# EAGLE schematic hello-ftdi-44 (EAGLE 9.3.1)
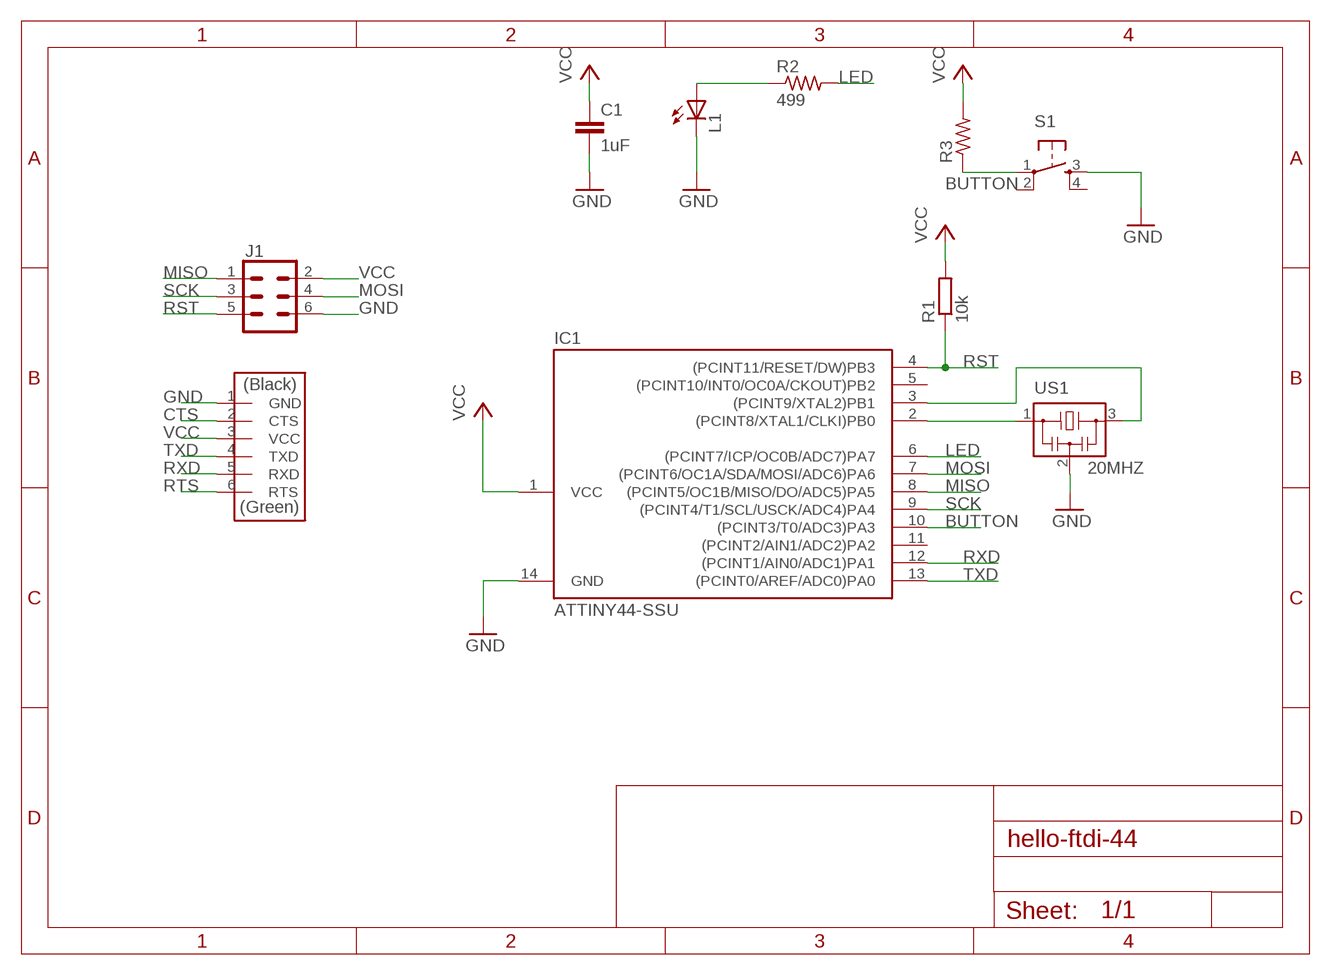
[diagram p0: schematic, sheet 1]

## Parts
C1  1uF  C-EUC1206  [C1206]
IC1  ATTINY44-SSU  [SOIC14]
J1  CONN_03X2SMT  [2X3_SMT_POSTS]
J2  FTDI-SMD-HEADER  [1X06SMD]
L1  LEDFAB1206  [LED1206FAB]
R1  10k  R-EU_M1206  [M1206]
R2  499  RES-US1206  [R1206]
R3  RES-US1206  [R1206]
S1  6MM_SWITCH6MM_SWITCH  [6MM_SWITCH]
US1  20MHZ  RESONATOR  [EFOBM]

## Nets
BUTTON: IC1.10((PCINT3/T0/ADC3)PA3) R3.1 S1.1(P)
CTS: J2.2(CTS)
GND: C1.2 IC1.14(GND) J1.6 J2.1(GND) L1.2(C) S1.3(S) US1.2
LED: IC1.6((PCINT7/ICP/OC0B/ADC7)PA7) R2.2
MISO: IC1.8((PCINT5/OC1B/MISO/DO/ADC5)PA5) J1.1
MOSI: IC1.7((PCINT6/OC1A/SDA/MOSI/ADC6)PA6) J1.4
N$1: L1.1(A) R2.1
N$7: IC1.2((PCINT8/XTAL1/CLKI)PB0) US1.1
N$8: IC1.3((PCINT9/XTAL2)PB1) US1.3
RST: IC1.4((PCINT11/RESET/DW)PB3) J1.5 R1.1
RTS: J2.6(RTS)
RXD: IC1.12((PCINT1/AIN0/ADC1)PA1) J2.5(RXD)
SCK: IC1.9((PCINT4/T1/SCL/USCK/ADC4)PA4) J1.3
TXD: IC1.13((PCINT0/AREF/ADC0)PA0) J2.4(TXD)
VCC: C1.1 IC1.1(VCC) J1.2 J2.3(VCC) R1.2 R3.2
Unconnected: IC1.5((PCINT10/INT0/OC0A/CKOUT)PB2) IC1.11((PCINT2/AIN1/ADC2)PA2) S1.2(P1) S1.4(S1)

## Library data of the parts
C1 = rcl:C-EU: CAPACITOR, European symbol
IC1 = fab:ATTINY44
J1 = SparkFun-Connectors:CONN_03X2: Multi connection point. Often used as Generic Header-pin footprint for 0.1 inch spaced/style header connections You can populate with any combo of single row headers, but if you'd like an exact match, check these: Header - 2x3 (Male, 0.1") (PRT-12807) Header - 2x3 (Female, 0.1") (PRT-13010) 2x3 Pin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; PROD_ID: CONN-11415
J2 = fab:FTDI-SMD-HEADER
L1 = fab:LED: LED
R1 = rcl:R-EU_: RESISTOR, European symbol
R2 R3 = fab:RES-US: Resistor (US Symbol)
S1 = fab:6MM_SWITCH: OMRON SWITCH
US1 = fab:RESONATOR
